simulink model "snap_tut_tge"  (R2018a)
settings: Solver=VariableStepDiscrete  StartTime=0.0  StopTime=50000  RelTol=1e-3
undefined symbols (not defined in the file): bad_frame, Bit, Both, bram, c, cnt_rst, core_rst, d, data, data_in, eof, eof_in, Falling, hex2dec, ip, ip_in, led, led_rx, led_tx, led_up, link_up, Location, Lower, Minimum_Area, notused, out, overrun, reg, Rising, ROACH2, sfp, SNAP, tx_full, tx_over, Unsigned, Upper, valid, valid_in, Width, xc7k160t
libraries: xbsIndex_r4 x1201, casper_library_misc x9, xps_library x5
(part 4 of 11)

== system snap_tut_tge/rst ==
  sim_1 : Inport
  sim_2 : Inport  Port=2
  convert1_1 : DataTypeConversion  OutDataTypeStr=fixdt('ufix1_En0')
  convert1_2 : DataTypeConversion  OutDataTypeStr=fixdt('ufix1_En0')
  convert2_1 : DataTypeConversion  OutDataTypeStr=fixdt('ufix1_En0')  ConvertRealWorld=Stored Integer (SI)
  convert2_2 : DataTypeConversion  OutDataTypeStr=fixdt('ufix1_En0')  ConvertRealWorld=Stored Integer (SI)
  gain_1 : Gain  Gain=2
  gain_2 : Gain
  io_delay : xbsIndex_r4/Delay  rst=off  infoeditControl=Selection of Reset will increase slice count due to use of real FFs and instead of SRLs  en=off  latency=0  reg_retiming=on  dbl_ovrd=off  block_type=delay
  sim_add : Sum  OutDataTypeStr=uint32
  slice_cnt_rst : xbsIndex_r4/Slice  nbits=1  boolean_output=on  mode=Lower Bit Location + Width  bit1=0  base1=MSB of Input  bit0=0  base0=LSB of Input  dbl_ovrd=off  block_type=slice
  slice_core_rst : xbsIndex_r4/Slice  nbits=1  boolean_output=on  mode=Lower Bit Location + Width  bit1=0  base1=MSB of Input  bit0=1  base0=LSB of Input  dbl_ovrd=off  block_type=slice
  snap_tut_tge_rst_user_data_out : xbsIndex_r4/Gateway In  gui_display_data_type=Fixed-point  arith_type=Unsigned  n_bits=32  bin_pt=0  preci_type=Single  exp_width=8  frac_width=24  rows=1  columns=1  quantization="Round  (unbiased: +/- Inf)"  overflow=Saturate  period=1  UseAsADC=off  ADCChannel='1'  interface=None  automatic_assignment=on  address_offset=hex2dec('00')  intf_name=''  intf_description=''  default_value=0  timing_constraint=None  locs_specified=off  LOCs={}  io_standard={}  inherit_from_input=off  hdl_port=on  dbl_ovrd=off  block_type=gatewayin
  in_core_rst : Outport
  in_cnt_rst : Outport  Port=2
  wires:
  snap_tut_tge_rst_user_data_out/1 -> io_delay/1
  sim_add/1 -> snap_tut_tge_rst_user_data_out/1
  sim_1/1 -> convert1_1/1
  convert1_1/1 -> convert2_1/1
  convert2_1/1 -> gain_1/1
  gain_1/1 -> sim_add/1
  io_delay/1 -> slice_core_rst/1, slice_cnt_rst/1
  slice_core_rst/1 -> in_core_rst/1
  sim_2/1 -> convert1_2/1
  convert1_2/1 -> convert2_2/1
  convert2_2/1 -> gain_2/1
  gain_2/1 -> sim_add/2
  slice_cnt_rst/1 -> in_cnt_rst/1

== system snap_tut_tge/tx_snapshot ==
  in_data : Inport
  in_valid : Inport  Port=2
  in_eof : Inport  Port=3
  we : Inport  Port=4
  trig : Inport  Port=5
  assert_data : xbsIndex_r4/Assert  assert_type=on  type_source=Explicitly  gui_display_data_type=Fixed-point  arith_type=Unsigned  n_bits=64  bin_pt=0  preci_type=Single  exp_width=8  frac_width=24  assert_rate=off  rate_source=Explicitly  period=1  output_port=on  block_type=assert
  assert_eof : xbsIndex_r4/Assert  assert_type=on  type_source=Explicitly  gui_display_data_type=Boolean  arith_type=Boolean  n_bits=1  bin_pt=0  preci_type=Single  exp_width=8  frac_width=24  assert_rate=off  rate_source=Explicitly  period=1  output_port=on  block_type=assert
  assert_valid : xbsIndex_r4/Assert  assert_type=on  type_source=Explicitly  gui_display_data_type=Boolean  arith_type=Boolean  n_bits=1  bin_pt=0  preci_type=Single  exp_width=8  frac_width=24  assert_rate=off  rate_source=Explicitly  period=1  output_port=on  block_type=assert
  buscreate : Subsystem  AncestorBlock=casper_library_flow_control/bus_create  mask(bus_create){inputNum=3}
      mask prompts: inputNum "Number of inputs:"
      mask init:
      | bus_create_init(gcb,...
      |     'inputNum', inputNum);
  ss : Subsystem  Tag=casper:snapshot  AncestorBlock=casper_library_scopes/snapshot  mask(snapshot){storage=bram, dram_dimm=2, dram_clock=250, nsamples=12, data_width=128, offset=off, circap=off, value=off, ext_arm=off, ext_circ=off, provide_outputs=off, use_dsp48=on}
      mask prompts: storage "Storage medium"; dram_dimm "DRAM dimm"; dram_clock "DRAM clock rate"; nsamples "Number of Samples (2^?)"; data_width "Data width"; offset "Start delay support"; circap "Circular capture support"; value "Extra value capture support"; ext_arm "External arm support"; ext_circ "External circular capture support"; provide_outputs "Provide outputs"; use_dsp48 "Use DSP48s to implement counters"
      mask help: Standard snap block, but with the following optional extras; 1) Optionally delay the fabric trigger by a user-specified number of valids. 2) Capture continuously after a trigger until a stop pulse is received. Data is captured into BRAM continuously, with old data being overwritten until a stop command is received. Then stop capturing when memory is filled. This enables you to get some data before and some data after the stop pulse. Use the 'tr_en_cnt' register to determine where you are in your vector. 'Addr' register's MSb now indicates 'busy capturing'. 3) Optionally capture a value on an i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
      mask init:
      | snapshot_init(gcb, ...
      |     'storage', storage, ...
      |     'dram_dimm', dram_dimm, ...
      |     'dram_clock', dram_clock, ...
      |     'nsamples', nsamples, ...
      |     'data_width', data_width, ...
      |     'offset', offset, ...
      |     'circap', circap, ...
      |     'value', value, ...
      |     'ext_arm', ext_arm, ...
      |     'ext_circ', ext_circ, ...
      |     'provide_outputs', 'off', ...
      |     'use_dsp48', use_dsp48);
  arm_out : Outport
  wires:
  ss/1(arm_out) -> arm_out/1
  buscreate/1(bus_out) -> ss/1(din)
  in_data/1 -> assert_data/1
  assert_data/1 -> buscreate/1(in1)
  in_valid/1 -> assert_valid/1
  assert_valid/1 -> buscreate/2(in2)
  in_eof/1 -> assert_eof/1
  assert_eof/1 -> buscreate/3(in3)
  we/1 -> ss/2(we)
  trig/1 -> ss/3(trig)

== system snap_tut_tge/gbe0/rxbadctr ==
  out_reg : Inport
  assert_reg : xbsIndex_r4/Assert  assert_type=on  type_source=Explicitly  gui_display_data_type=Fixed-point  arith_type=Unsigned  n_bits=32  bin_pt=0  preci_type=Single  exp_width=8  frac_width=24  assert_rate=off  rate_source=Explicitly  period=1  output_port=on  block_type=assert
  cast_gw : xbsIndex_r4/Convert  gui_display_data_type=Fixed-point  arith_type=Unsigned  n_bits=32  bin_pt=0  float_type=Single  exp_bits=8  fraction_bits=24  quantization=Truncate  overflow=Wrap  en=off  latency=1  pipeline=off  dbl_ovrd=off  block_type=convert
  io_delay : xbsIndex_r4/Delay  rst=off  infoeditControl=Selection of Reset will increase slice count due to use of real FFs and instead of SRLs  en=off  latency=1  reg_retiming=on  dbl_ovrd=off  block_type=delay
  reint1 : xbsIndex_r4/Reinterpret  force_arith_type=on  arith_type=Unsigned  force_bin_pt=on  bin_pt=0  block_type=reinterpret
  sim_out : Terminator
  snap_tut_tge_gbe0_rxbadctr_user_data_in : xbsIndex_r4/Gateway Out  inherit_from_input=off  hdl_port=on  rows=1  columns=1  UseAsDAC=off  DACChannel='1'  interface=None  automatic_assignment=on  address_offset=hex2dec('00')  intf_name=''  intf_description=''  timing_constraint=None  locs_specified=off  LOCs={}  io_standard={}  block_type=gatewayout
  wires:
  io_delay/1 -> cast_gw/1
  cast_gw/1 -> snap_tut_tge_gbe0_rxbadctr_user_data_in/1
  snap_tut_tge_gbe0_rxbadctr_user_data_in/1 -> sim_out/1
  out_reg/1 -> assert_reg/1
  assert_reg/1 -> reint1/1
  reint1/1 -> io_delay/1

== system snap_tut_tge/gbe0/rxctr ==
  out_reg : Inport
  assert_reg : xbsIndex_r4/Assert  assert_type=on  type_source=Explicitly  gui_display_data_type=Fixed-point  arith_type=Unsigned  n_bits=32  bin_pt=0  preci_type=Single  exp_width=8  frac_width=24  assert_rate=off  rate_source=Explicitly  period=1  output_port=on  block_type=assert
  cast_gw : xbsIndex_r4/Convert  gui_display_data_type=Fixed-point  arith_type=Unsigned  n_bits=32  bin_pt=0  float_type=Single  exp_bits=8  fraction_bits=24  quantization=Truncate  overflow=Wrap  en=off  latency=1  pipeline=off  dbl_ovrd=off  block_type=convert
  io_delay : xbsIndex_r4/Delay  rst=off  infoeditControl=Selection of Reset will increase slice count due to use of real FFs and instead of SRLs  en=off  latency=1  reg_retiming=on  dbl_ovrd=off  block_type=delay
  reint1 : xbsIndex_r4/Reinterpret  force_arith_type=on  arith_type=Unsigned  force_bin_pt=on  bin_pt=0  block_type=reinterpret
  sim_out : Terminator
  snap_tut_tge_gbe0_rxctr_user_data_in : xbsIndex_r4/Gateway Out  inherit_from_input=off  hdl_port=on  rows=1  columns=1  UseAsDAC=off  DACChannel='1'  interface=None  automatic_assignment=on  address_offset=hex2dec('00')  intf_name=''  intf_description=''  timing_constraint=None  locs_specified=off  LOCs={}  io_standard={}  block_type=gatewayout
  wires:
  io_delay/1 -> cast_gw/1
  cast_gw/1 -> snap_tut_tge_gbe0_rxctr_user_data_in/1
  snap_tut_tge_gbe0_rxctr_user_data_in/1 -> sim_out/1
  out_reg/1 -> assert_reg/1
  assert_reg/1 -> reint1/1
  reint1/1 -> io_delay/1

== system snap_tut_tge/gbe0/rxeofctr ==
  out_reg : Inport
  assert_reg : xbsIndex_r4/Assert  assert_type=on  type_source=Explicitly  gui_display_data_type=Fixed-point  arith_type=Unsigned  n_bits=32  bin_pt=0  preci_type=Single  exp_width=8  frac_width=24  assert_rate=off  rate_source=Explicitly  period=1  output_port=on  block_type=assert
  cast_gw : xbsIndex_r4/Convert  gui_display_data_type=Fixed-point  arith_type=Unsigned  n_bits=32  bin_pt=0  float_type=Single  exp_bits=8  fraction_bits=24  quantization=Truncate  overflow=Wrap  en=off  latency=1  pipeline=off  dbl_ovrd=off  block_type=convert
  io_delay : xbsIndex_r4/Delay  rst=off  infoeditControl=Selection of Reset will increase slice count due to use of real FFs and instead of SRLs  en=off  latency=1  reg_retiming=on  dbl_ovrd=off  block_type=delay
  reint1 : xbsIndex_r4/Reinterpret  force_arith_type=on  arith_type=Unsigned  force_bin_pt=on  bin_pt=0  block_type=reinterpret
  sim_out : Terminator
  snap_tut_tge_gbe0_rxeofctr_user_data_in : xbsIndex_r4/Gateway Out  inherit_from_input=off  hdl_port=on  rows=1  columns=1  UseAsDAC=off  DACChannel='1'  interface=None  automatic_assignment=on  address_offset=hex2dec('00')  intf_name=''  intf_description=''  timing_constraint=None  locs_specified=off  LOCs={}  io_standard={}  block_type=gatewayout
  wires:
  io_delay/1 -> cast_gw/1
  cast_gw/1 -> snap_tut_tge_gbe0_rxeofctr_user_data_in/1
  snap_tut_tge_gbe0_rxeofctr_user_data_in/1 -> sim_out/1
  out_reg/1 -> assert_reg/1
  assert_reg/1 -> reint1/1
  reint1/1 -> io_delay/1

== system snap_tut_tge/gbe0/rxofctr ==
  out_reg : Inport
  assert_reg : xbsIndex_r4/Assert  assert_type=on  type_source=Explicitly  gui_display_data_type=Fixed-point  arith_type=Unsigned  n_bits=32  bin_pt=0  preci_type=Single  exp_width=8  frac_width=24  assert_rate=off  rate_source=Explicitly  period=1  output_port=on  block_type=assert
  cast_gw : xbsIndex_r4/Convert  gui_display_data_type=Fixed-point  arith_type=Unsigned  n_bits=32  bin_pt=0  float_type=Single  exp_bits=8  fraction_bits=24  quantization=Truncate  overflow=Wrap  en=off  latency=1  pipeline=off  dbl_ovrd=off  block_type=convert
  io_delay : xbsIndex_r4/Delay  rst=off  infoeditControl=Selection of Reset will increase slice count due to use of real FFs and instead of SRLs  en=off  latency=1  reg_retiming=on  dbl_ovrd=off  block_type=delay
  reint1 : xbsIndex_r4/Reinterpret  force_arith_type=on  arith_type=Unsigned  force_bin_pt=on  bin_pt=0  block_type=reinterpret
  sim_out : Terminator
  snap_tut_tge_gbe0_rxofctr_user_data_in : xbsIndex_r4/Gateway Out  inherit_from_input=off  hdl_port=on  rows=1  columns=1  UseAsDAC=off  DACChannel='1'  interface=None  automatic_assignment=on  address_offset=hex2dec('00')  intf_name=''  intf_description=''  timing_constraint=None  locs_specified=off  LOCs={}  io_standard={}  block_type=gatewayout
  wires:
  io_delay/1 -> cast_gw/1
  cast_gw/1 -> snap_tut_tge_gbe0_rxofctr_user_data_in/1
  snap_tut_tge_gbe0_rxofctr_user_data_in/1 -> sim_out/1
  out_reg/1 -> assert_reg/1
  assert_reg/1 -> reint1/1
  reint1/1 -> io_delay/1

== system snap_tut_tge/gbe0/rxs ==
  in_led_up : Inport
  in_led_rx : Inport  Port=2
  in_data_in : Inport  Port=3
  in_valid_in : Inport  Port=4
  in_ip_in : Inport  Port=5
  in_eof_in : Inport  Port=6
  in_bad_frame : Inport  Port=7
  in_overrun : Inport  Port=8
  we : Inport  Port=9
  trig : Inport  Port=10
  assert_bad_frame : xbsIndex_r4/Assert  assert_type=on  type_source=Explicitly  gui_display_data_type=Boolean  arith_type=Boolean  n_bits=1  bin_pt=0  preci_type=Single  exp_width=8  frac_width=24  assert_rate=off  rate_source=Explicitly  period=1  output_port=on  block_type=assert
  assert_data_in : xbsIndex_r4/Assert  assert_type=on  type_source=Explicitly  gui_display_data_type=Fixed-point  arith_type=Unsigned  n_bits=64  bin_pt=0  preci_type=Single  exp_width=8  frac_width=24  assert_rate=off  rate_source=Explicitly  period=1  output_port=on  block_type=assert
  assert_eof_in : xbsIndex_r4/Assert  assert_type=on  type_source=Explicitly  gui_display_data_type=Boolean  arith_type=Boolean  n_bits=1  bin_pt=0  preci_type=Single  exp_width=8  frac_width=24  assert_rate=off  rate_source=Explicitly  period=1  output_port=on  block_type=assert
  assert_ip_in : xbsIndex_r4/Assert  assert_type=on  type_source=Explicitly  gui_display_data_type=Fixed-point  arith_type=Unsigned  n_bits=32  bin_pt=0  preci_type=Single  exp_width=8  frac_width=24  assert_rate=off  rate_source=Explicitly  period=1  output_port=on  block_type=assert
  assert_led_rx : xbsIndex_r4/Assert  assert_type=on  type_source=Explicitly  gui_display_data_type=Boolean  arith_type=Boolean  n_bits=1  bin_pt=0  preci_type=Single  exp_width=8  frac_width=24  assert_rate=off  rate_source=Explicitly  period=1  output_port=on  block_type=assert
  assert_led_up : xbsIndex_r4/Assert  assert_type=on  type_source=Explicitly  gui_display_data_type=Boolean  arith_type=Boolean  n_bits=1  bin_pt=0  preci_type=Single  exp_width=8  frac_width=24  assert_rate=off  rate_source=Explicitly  period=1  output_port=on  block_type=assert
  assert_overrun : xbsIndex_r4/Assert  assert_type=on  type_source=Explicitly  gui_display_data_type=Boolean  arith_type=Boolean  n_bits=1  bin_pt=0  preci_type=Single  exp_width=8  frac_width=24  assert_rate=off  rate_source=Explicitly  period=1  output_port=on  block_type=assert
  assert_valid_in : xbsIndex_r4/Assert  assert_type=on  type_source=Explicitly  gui_display_data_type=Boolean  arith_type=Boolean  n_bits=1  bin_pt=0  preci_type=Single  exp_width=8  frac_width=24  assert_rate=off  rate_source=Explicitly  period=1  output_port=on  block_type=assert
  buscreate : Subsystem  AncestorBlock=casper_library_flow_control/bus_create  mask(bus_create){inputNum=8}
      mask prompts: inputNum "Number of inputs:"
      mask init:
      | bus_create_init(gcb,...
      |     'inputNum', inputNum);
  io_delay : Subsystem  AncestorBlock=casper_library_delays/pipeline  mask(pipeline){csp_latency=5}
      mask prompts: csp_latency "Latency"
      mask help: An explicitly laid-out delay line to avoid mapping to SRL16s for use in pipelining to help achieve timing closure.
      mask init:
      | pipeline_init(gcb,'latency',csp_latency);
  ss : Subsystem  Tag=casper:snapshot  AncestorBlock=casper_library_scopes/snapshot  mask(snapshot){storage=bram, dram_dimm=2, dram_clock=250, nsamples=13, data_width=128, offset=off, circap=off, value=off, ext_arm=off, ext_circ=off, provide_outputs=off, use_dsp48=on}
      mask prompts: storage "Storage medium"; dram_dimm "DRAM dimm"; dram_clock "DRAM clock rate"; nsamples "Number of Samples (2^?)"; data_width "Data width"; offset "Start delay support"; circap "Circular capture support"; value "Extra value capture support"; ext_arm "External arm support"; ext_circ "External circular capture support"; provide_outputs "Provide outputs"; use_dsp48 "Use DSP48s to implement counters"
      mask help: Standard snap block, but with the following optional extras; 1) Optionally delay the fabric trigger by a user-specified number of valids. 2) Capture continuously after a trigger until a stop pulse is received. Data is captured into BRAM continuously, with old data being overwritten until a stop command is received. Then stop capturing when memory is filled. This enables you to get some data before and some data after the stop pulse. Use the 'tr_en_cnt' register to determine where you are in your vector. 'Addr' register's MSb now indicates 'busy capturing'. 3) Optionally capture a value on an i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
      mask init:
      | snapshot_init(gcb, ...
      |     'storage', storage, ...
      |     'dram_dimm', dram_dimm, ...
      |     'dram_clock', dram_clock, ...
      |     'nsamples', nsamples, ...
      |     'data_width', data_width, ...
      |     'offset', offset, ...
      |     'circap', circap, ...
      |     'value', value, ...
      |     'ext_arm', ext_arm, ...
      |     'ext_circ', ext_circ, ...
      |     'provide_outputs', 'off', ...
      |     'use_dsp48', use_dsp48);
  trig_delay : Subsystem  AncestorBlock=casper_library_delays/pipeline  mask(pipeline){csp_latency=5}
      mask prompts: csp_latency "Latency"
      mask help: An explicitly laid-out delay line to avoid mapping to SRL16s for use in pipelining to help achieve timing closure.
      mask init:
      | pipeline_init(gcb,'latency',csp_latency);
  we_delay : Subsystem  AncestorBlock=casper_library_delays/pipeline  mask(pipeline){csp_latency=5}
      mask prompts: csp_latency "Latency"
      mask help: An explicitly laid-out delay line to avoid mapping to SRL16s for use in pipelining to help achieve timing closure.
      mask init:
      | pipeline_init(gcb,'latency',csp_latency);
  arm_out : Outport
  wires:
  ss/1(arm_out) -> arm_out/1
  buscreate/1(bus_out) -> io_delay/1(d)
  io_delay/1(q) -> ss/1(din)
  in_led_up/1 -> assert_led_up/1
  assert_led_up/1 -> buscreate/1(in1)
  in_led_rx/1 -> assert_led_rx/1
  assert_led_rx/1 -> buscreate/2(in2)
  in_data_in/1 -> assert_data_in/1
  assert_data_in/1 -> buscreate/3(in3)
  in_valid_in/1 -> assert_valid_in/1
  assert_valid_in/1 -> buscreate/4(in4)
  in_ip_in/1 -> assert_ip_in/1
  assert_ip_in/1 -> buscreate/5(in5)
  in_eof_in/1 -> assert_eof_in/1
  assert_eof_in/1 -> buscreate/6(in6)
  in_bad_frame/1 -> assert_bad_frame/1
  assert_bad_frame/1 -> buscreate/7(in7)
  in_overrun/1 -> assert_overrun/1
  assert_overrun/1 -> buscreate/8(in8)
  we/1 -> we_delay/1(d)
  we_delay/1(q) -> ss/2(we)
  trig/1 -> trig_delay/1(d)
  trig_delay/1(q) -> ss/3(trig)

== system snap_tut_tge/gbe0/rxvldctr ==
  out_reg : Inport
  assert_reg : xbsIndex_r4/Assert  assert_type=on  type_source=Explicitly  gui_display_data_type=Fixed-point  arith_type=Unsigned  n_bits=32  bin_pt=0  preci_type=Single  exp_width=8  frac_width=24  assert_rate=off  rate_source=Explicitly  period=1  output_port=on  block_type=assert
  cast_gw : xbsIndex_r4/Convert  gui_display_data_type=Fixed-point  arith_type=Unsigned  n_bits=32  bin_pt=0  float_type=Single  exp_bits=8  fraction_bits=24  quantization=Truncate  overflow=Wrap  en=off  latency=1  pipeline=off  dbl_ovrd=off  block_type=convert
  io_delay : xbsIndex_r4/Delay  rst=off  infoeditControl=Selection of Reset will increase slice count due to use of real FFs and instead of SRLs  en=off  latency=1  reg_retiming=on  dbl_ovrd=off  block_type=delay
  reint1 : xbsIndex_r4/Reinterpret  force_arith_type=on  arith_type=Unsigned  force_bin_pt=on  bin_pt=0  block_type=reinterpret
  sim_out : Terminator
  snap_tut_tge_gbe0_rxvldctr_user_data_in : xbsIndex_r4/Gateway Out  inherit_from_input=off  hdl_port=on  rows=1  columns=1  UseAsDAC=off  DACChannel='1'  interface=None  automatic_assignment=on  address_offset=hex2dec('00')  intf_name=''  intf_description=''  timing_constraint=None  locs_specified=off  LOCs={}  io_standard={}  block_type=gatewayout
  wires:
  io_delay/1 -> cast_gw/1
  cast_gw/1 -> snap_tut_tge_gbe0_rxvldctr_user_data_in/1
  snap_tut_tge_gbe0_rxvldctr_user_data_in/1 -> sim_out/1
  out_reg/1 -> assert_reg/1
  assert_reg/1 -> reint1/1
  reint1/1 -> io_delay/1

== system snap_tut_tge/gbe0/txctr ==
  out_reg : Inport
  assert_reg : xbsIndex_r4/Assert  assert_type=on  type_source=Explicitly  gui_display_data_type=Fixed-point  arith_type=Unsigned  n_bits=32  bin_pt=0  preci_type=Single  exp_width=8  frac_width=24  assert_rate=off  rate_source=Explicitly  period=1  output_port=on  block_type=assert
  cast_gw : xbsIndex_r4/Convert  gui_display_data_type=Fixed-point  arith_type=Unsigned  n_bits=32  bin_pt=0  float_type=Single  exp_bits=8  fraction_bits=24  quantization=Truncate  overflow=Wrap  en=off  latency=1  pipeline=off  dbl_ovrd=off  block_type=convert
  io_delay : xbsIndex_r4/Delay  rst=off  infoeditControl=Selection of Reset will increase slice count due to use of real FFs and instead of SRLs  en=off  latency=1  reg_retiming=on  dbl_ovrd=off  block_type=delay
  reint1 : xbsIndex_r4/Reinterpret  force_arith_type=on  arith_type=Unsigned  force_bin_pt=on  bin_pt=0  block_type=reinterpret
  sim_out : Terminator
  snap_tut_tge_gbe0_txctr_user_data_in : xbsIndex_r4/Gateway Out  inherit_from_input=off  hdl_port=on  rows=1  columns=1  UseAsDAC=off  DACChannel='1'  interface=None  automatic_assignment=on  address_offset=hex2dec('00')  intf_name=''  intf_description=''  timing_constraint=None  locs_specified=off  LOCs={}  io_standard={}  block_type=gatewayout
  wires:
  io_delay/1 -> cast_gw/1
  cast_gw/1 -> snap_tut_tge_gbe0_txctr_user_data_in/1
  snap_tut_tge_gbe0_txctr_user_data_in/1 -> sim_out/1
  out_reg/1 -> assert_reg/1
  assert_reg/1 -> reint1/1
  reint1/1 -> io_delay/1

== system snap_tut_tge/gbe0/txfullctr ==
  out_reg : Inport
  assert_reg : xbsIndex_r4/Assert  assert_type=on  type_source=Explicitly  gui_display_data_type=Fixed-point  arith_type=Unsigned  n_bits=32  bin_pt=0  preci_type=Single  exp_width=8  frac_width=24  assert_rate=off  rate_source=Explicitly  period=1  output_port=on  block_type=assert
  cast_gw : xbsIndex_r4/Convert  gui_display_data_type=Fixed-point  arith_type=Unsigned  n_bits=32  bin_pt=0  float_type=Single  exp_bits=8  fraction_bits=24  quantization=Truncate  overflow=Wrap  en=off  latency=1  pipeline=off  dbl_ovrd=off  block_type=convert
  io_delay : xbsIndex_r4/Delay  rst=off  infoeditControl=Selection of Reset will increase slice count due to use of real FFs and instead of SRLs  en=off  latency=1  reg_retiming=on  dbl_ovrd=off  block_type=delay
  reint1 : xbsIndex_r4/Reinterpret  force_arith_type=on  arith_type=Unsigned  force_bin_pt=on  bin_pt=0  block_type=reinterpret
  sim_out : Terminator
  snap_tut_tge_gbe0_txfullctr_user_data_in : xbsIndex_r4/Gateway Out  inherit_from_input=off  hdl_port=on  rows=1  columns=1  UseAsDAC=off  DACChannel='1'  interface=None  automatic_assignment=on  address_offset=hex2dec('00')  intf_name=''  intf_description=''  timing_constraint=None  locs_specified=off  LOCs={}  io_standard={}  block_type=gatewayout
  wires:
  io_delay/1 -> cast_gw/1
  cast_gw/1 -> snap_tut_tge_gbe0_txfullctr_user_data_in/1
  snap_tut_tge_gbe0_txfullctr_user_data_in/1 -> sim_out/1
  out_reg/1 -> assert_reg/1
  assert_reg/1 -> reint1/1
  reint1/1 -> io_delay/1

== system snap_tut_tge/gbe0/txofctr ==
  out_reg : Inport
  assert_reg : xbsIndex_r4/Assert  assert_type=on  type_source=Explicitly  gui_display_data_type=Fixed-point  arith_type=Unsigned  n_bits=32  bin_pt=0  preci_type=Single  exp_width=8  frac_width=24  assert_rate=off  rate_source=Explicitly  period=1  output_port=on  block_type=assert
  cast_gw : xbsIndex_r4/Convert  gui_display_data_type=Fixed-point  arith_type=Unsigned  n_bits=32  bin_pt=0  float_type=Single  exp_bits=8  fraction_bits=24  quantization=Truncate  overflow=Wrap  en=off  latency=1  pipeline=off  dbl_ovrd=off  block_type=convert
  io_delay : xbsIndex_r4/Delay  rst=off  infoeditControl=Selection of Reset will increase slice count due to use of real FFs and instead of SRLs  en=off  latency=1  reg_retiming=on  dbl_ovrd=off  block_type=delay
  reint1 : xbsIndex_r4/Reinterpret  force_arith_type=on  arith_type=Unsigned  force_bin_pt=on  bin_pt=0  block_type=reinterpret
  sim_out : Terminator
  snap_tut_tge_gbe0_txofctr_user_data_in : xbsIndex_r4/Gateway Out  inherit_from_input=off  hdl_port=on  rows=1  columns=1  UseAsDAC=off  DACChannel='1'  interface=None  automatic_assignment=on  address_offset=hex2dec('00')  intf_name=''  intf_description=''  timing_constraint=None  locs_specified=off  LOCs={}  io_standard={}  block_type=gatewayout
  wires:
  io_delay/1 -> cast_gw/1
  cast_gw/1 -> snap_tut_tge_gbe0_txofctr_user_data_in/1
  snap_tut_tge_gbe0_txofctr_user_data_in/1 -> sim_out/1
  out_reg/1 -> assert_reg/1
  assert_reg/1 -> reint1/1
  reint1/1 -> io_delay/1

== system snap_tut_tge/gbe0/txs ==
  in_link_up : Inport
  in_led_tx : Inport  Port=2
  in_tx_full : Inport  Port=3
  in_tx_over : Inport  Port=4
  in_valid : Inport  Port=5
  in_eof : Inport  Port=6
  in_data : Inport  Port=7
  in_ip : Inport  Port=8
  we : Inport  Port=9
  trig : Inport  Port=10
  assert_data : xbsIndex_r4/Assert  assert_type=on  type_source=Explicitly  gui_display_data_type=Fixed-point  arith_type=Unsigned  n_bits=64  bin_pt=0  preci_type=Single  exp_width=8  frac_width=24  assert_rate=off  rate_source=Explicitly  period=1  output_port=on  block_type=assert
  assert_eof : xbsIndex_r4/Assert  assert_type=on  type_source=Explicitly  gui_display_data_type=Boolean  arith_type=Boolean  n_bits=1  bin_pt=0  preci_type=Single  exp_width=8  frac_width=24  assert_rate=off  rate_source=Explicitly  period=1  output_port=on  block_type=assert
  assert_ip : xbsIndex_r4/Assert  assert_type=on  type_source=Explicitly  gui_display_data_type=Fixed-point  arith_type=Unsigned  n_bits=32  bin_pt=0  preci_type=Single  exp_width=8  frac_width=24  assert_rate=off  rate_source=Explicitly  period=1  output_port=on  block_type=assert
  assert_led_tx : xbsIndex_r4/Assert  assert_type=on  type_source=Explicitly  gui_display_data_type=Boolean  arith_type=Boolean  n_bits=1  bin_pt=0  preci_type=Single  exp_width=8  frac_width=24  assert_rate=off  rate_source=Explicitly  period=1  output_port=on  block_type=assert
  assert_link_up : xbsIndex_r4/Assert  assert_type=on  type_source=Explicitly  gui_display_data_type=Boolean  arith_type=Boolean  n_bits=1  bin_pt=0  preci_type=Single  exp_width=8  frac_width=24  assert_rate=off  rate_source=Explicitly  period=1  output_port=on  block_type=assert
  assert_tx_full : xbsIndex_r4/Assert  assert_type=on  type_source=Explicitly  gui_display_data_type=Boolean  arith_type=Boolean  n_bits=1  bin_pt=0  preci_type=Single  exp_width=8  frac_width=24  assert_rate=off  rate_source=Explicitly  period=1  output_port=on  block_type=assert
  assert_tx_over : xbsIndex_r4/Assert  assert_type=on  type_source=Explicitly  gui_display_data_type=Boolean  arith_type=Boolean  n_bits=1  bin_pt=0  preci_type=Single  exp_width=8  frac_width=24  assert_rate=off  rate_source=Explicitly  period=1  output_port=on  block_type=assert
  assert_valid : xbsIndex_r4/Assert  assert_type=on  type_source=Explicitly  gui_display_data_type=Boolean  arith_type=Boolean  n_bits=1  bin_pt=0  preci_type=Single  exp_width=8  frac_width=24  assert_rate=off  rate_source=Explicitly  period=1  output_port=on  block_type=assert
  buscreate : Subsystem  AncestorBlock=casper_library_flow_control/bus_create  mask(bus_create){inputNum=8}
      mask prompts: inputNum "Number of inputs:"
      mask init:
      | bus_create_init(gcb,...
      |     'inputNum', inputNum);
  io_delay : Subsystem  AncestorBlock=casper_library_delays/pipeline  mask(pipeline){csp_latency=5}
      mask prompts: csp_latency "Latency"
      mask help: An explicitly laid-out delay line to avoid mapping to SRL16s for use in pipelining to help achieve timing closure.
      mask init:
      | pipeline_init(gcb,'latency',csp_latency);
  ss : Subsystem  Tag=casper:snapshot  AncestorBlock=casper_library_scopes/snapshot  mask(snapshot){storage=bram, dram_dimm=2, dram_clock=250, nsamples=13, data_width=128, offset=off, circap=off, value=off, ext_arm=off, ext_circ=off, provide_outputs=off, use_dsp48=on}
      mask prompts: storage "Storage medium"; dram_dimm "DRAM dimm"; dram_clock "DRAM clock rate"; nsamples "Number of Samples (2^?)"; data_width "Data width"; offset "Start delay support"; circap "Circular capture support"; value "Extra value capture support"; ext_arm "External arm support"; ext_circ "External circular capture support"; provide_outputs "Provide outputs"; use_dsp48 "Use DSP48s to implement counters"
      mask help: Standard snap block, but with the following optional extras; 1) Optionally delay the fabric trigger by a user-specified number of valids. 2) Capture continuously after a trigger until a stop pulse is received. Data is captured into BRAM continuously, with old data being overwritten until a stop command is received. Then stop capturing when memory is filled. This enables you to get some data before and some data after the stop pulse. Use the 'tr_en_cnt' register to determine where you are in your vector. 'Addr' register's MSb now indicates 'busy capturing'. 3) Optionally capture a value on an i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
      mask init:
      | snapshot_init(gcb, ...
      |     'storage', storage, ...
      |     'dram_dimm', dram_dimm, ...
      |     'dram_clock', dram_clock, ...
      |     'nsamples', nsamples, ...
      |     'data_width', data_width, ...
      |     'offset', offset, ...
      |     'circap', circap, ...
      |     'value', value, ...
      |     'ext_arm', ext_arm, ...
      |     'ext_circ', ext_circ, ...
      |     'provide_outputs', 'off', ...
      |     'use_dsp48', use_dsp48);
  trig_delay : Subsystem  AncestorBlock=casper_library_delays/pipeline  mask(pipeline){csp_latency=5}
      mask prompts: csp_latency "Latency"
      mask help: An explicitly laid-out delay line to avoid mapping to SRL16s for use in pipelining to help achieve timing closure.
      mask init:
      | pipeline_init(gcb,'latency',csp_latency);
  we_delay : Subsystem  AncestorBlock=casper_library_delays/pipeline  mask(pipeline){csp_latency=5}
      mask prompts: csp_latency "Latency"
      mask help: An explicitly laid-out delay line to avoid mapping to SRL16s for use in pipelining to help achieve timing closure.
      mask init:
      | pipeline_init(gcb,'latency',csp_latency);
  arm_out : Outport
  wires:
  ss/1(arm_out) -> arm_out/1
  buscreate/1(bus_out) -> io_delay/1(d)
  io_delay/1(q) -> ss/1(din)
  in_link_up/1 -> assert_link_up/1
  assert_link_up/1 -> buscreate/1(in1)
  in_led_tx/1 -> assert_led_tx/1
  assert_led_tx/1 -> buscreate/2(in2)
  in_tx_full/1 -> assert_tx_full/1
  assert_tx_full/1 -> buscreate/3(in3)
  in_tx_over/1 -> assert_tx_over/1
  assert_tx_over/1 -> buscreate/4(in4)
  in_valid/1 -> assert_valid/1
  assert_valid/1 -> buscreate/5(in5)
  in_eof/1 -> assert_eof/1
  assert_eof/1 -> buscreate/6(in6)
  in_data/1 -> assert_data/1
  assert_data/1 -> buscreate/7(in7)
  in_ip/1 -> assert_ip/1
  assert_ip/1 -> buscreate/8(in8)
  we/1 -> we_delay/1(d)
  we_delay/1(q) -> ss/2(we)
  trig/1 -> trig_delay/1(d)
  trig_delay/1(q) -> ss/3(trig)

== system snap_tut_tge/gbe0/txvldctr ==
  out_reg : Inport
  assert_reg : xbsIndex_r4/Assert  assert_type=on  type_source=Explicitly  gui_display_data_type=Fixed-point  arith_type=Unsigned  n_bits=32  bin_pt=0  preci_type=Single  exp_width=8  frac_width=24  assert_rate=off  rate_source=Explicitly  period=1  output_port=on  block_type=assert
  cast_gw : xbsIndex_r4/Convert  gui_display_data_type=Fixed-point  arith_type=Unsigned  n_bits=32  bin_pt=0  float_type=Single  exp_bits=8  fraction_bits=24  quantization=Truncate  overflow=Wrap  en=off  latency=1  pipeline=off  dbl_ovrd=off  block_type=convert
  io_delay : xbsIndex_r4/Delay  rst=off  infoeditControl=Selection of Reset will increase slice count due to use of real FFs and instead of SRLs  en=off  latency=1  reg_retiming=on  dbl_ovrd=off  block_type=delay
  reint1 : xbsIndex_r4/Reinterpret  force_arith_type=on  arith_type=Unsigned  force_bin_pt=on  bin_pt=0  block_type=reinterpret
  sim_out : Terminator
  snap_tut_tge_gbe0_txvldctr_user_data_in : xbsIndex_r4/Gateway Out  inherit_from_input=off  hdl_port=on  rows=1  columns=1  UseAsDAC=off  DACChannel='1'  interface=None  automatic_assignment=on  address_offset=hex2dec('00')  intf_name=''  intf_description=''  timing_constraint=None  locs_specified=off  LOCs={}  io_standard={}  block_type=gatewayout
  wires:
  io_delay/1 -> cast_gw/1
  cast_gw/1 -> snap_tut_tge_gbe0_txvldctr_user_data_in/1
  snap_tut_tge_gbe0_txvldctr_user_data_in/1 -> sim_out/1
  out_reg/1 -> assert_reg/1
  assert_reg/1 -> reint1/1
  reint1/1 -> io_delay/1

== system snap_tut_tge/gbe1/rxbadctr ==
  out_reg : Inport
  assert_reg : xbsIndex_r4/Assert  assert_type=on  type_source=Explicitly  gui_display_data_type=Fixed-point  arith_type=Unsigned  n_bits=32  bin_pt=0  preci_type=Single  exp_width=8  frac_width=24  assert_rate=off  rate_source=Explicitly  period=1  output_port=on  block_type=assert
  cast_gw : xbsIndex_r4/Convert  gui_display_data_type=Fixed-point  arith_type=Unsigned  n_bits=32  bin_pt=0  float_type=Single  exp_bits=8  fraction_bits=24  quantization=Truncate  overflow=Wrap  en=off  latency=1  pipeline=off  dbl_ovrd=off  block_type=convert
  io_delay : xbsIndex_r4/Delay  rst=off  infoeditControl=Selection of Reset will increase slice count due to use of real FFs and instead of SRLs  en=off  latency=1  reg_retiming=on  dbl_ovrd=off  block_type=delay
  reint1 : xbsIndex_r4/Reinterpret  force_arith_type=on  arith_type=Unsigned  force_bin_pt=on  bin_pt=0  block_type=reinterpret
  sim_out : Terminator
  snap_tut_tge_gbe1_rxbadctr_user_data_in : xbsIndex_r4/Gateway Out  inherit_from_input=off  hdl_port=on  rows=1  columns=1  UseAsDAC=off  DACChannel='1'  interface=None  automatic_assignment=on  address_offset=hex2dec('00')  intf_name=''  intf_description=''  timing_constraint=None  locs_specified=off  LOCs={}  io_standard={}  block_type=gatewayout
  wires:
  io_delay/1 -> cast_gw/1
  cast_gw/1 -> snap_tut_tge_gbe1_rxbadctr_user_data_in/1
  snap_tut_tge_gbe1_rxbadctr_user_data_in/1 -> sim_out/1
  out_reg/1 -> assert_reg/1
  assert_reg/1 -> reint1/1
  reint1/1 -> io_delay/1

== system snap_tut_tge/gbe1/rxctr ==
  out_reg : Inport
  assert_reg : xbsIndex_r4/Assert  assert_type=on  type_source=Explicitly  gui_display_data_type=Fixed-point  arith_type=Unsigned  n_bits=32  bin_pt=0  preci_type=Single  exp_width=8  frac_width=24  assert_rate=off  rate_source=Explicitly  period=1  output_port=on  block_type=assert
  cast_gw : xbsIndex_r4/Convert  gui_display_data_type=Fixed-point  arith_type=Unsigned  n_bits=32  bin_pt=0  float_type=Single  exp_bits=8  fraction_bits=24  quantization=Truncate  overflow=Wrap  en=off  latency=1  pipeline=off  dbl_ovrd=off  block_type=convert
  io_delay : xbsIndex_r4/Delay  rst=off  infoeditControl=Selection of Reset will increase slice count due to use of real FFs and instead of SRLs  en=off  latency=1  reg_retiming=on  dbl_ovrd=off  block_type=delay
  reint1 : xbsIndex_r4/Reinterpret  force_arith_type=on  arith_type=Unsigned  force_bin_pt=on  bin_pt=0  block_type=reinterpret
  sim_out : Terminator
  snap_tut_tge_gbe1_rxctr_user_data_in : xbsIndex_r4/Gateway Out  inherit_from_input=off  hdl_port=on  rows=1  columns=1  UseAsDAC=off  DACChannel='1'  interface=None  automatic_assignment=on  address_offset=hex2dec('00')  intf_name=''  intf_description=''  timing_constraint=None  locs_specified=off  LOCs={}  io_standard={}  block_type=gatewayout
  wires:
  io_delay/1 -> cast_gw/1
  cast_gw/1 -> snap_tut_tge_gbe1_rxctr_user_data_in/1
  snap_tut_tge_gbe1_rxctr_user_data_in/1 -> sim_out/1
  out_reg/1 -> assert_reg/1
  assert_reg/1 -> reint1/1
  reint1/1 -> io_delay/1

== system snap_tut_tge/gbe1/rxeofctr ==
  out_reg : Inport
  assert_reg : xbsIndex_r4/Assert  assert_type=on  type_source=Explicitly  gui_display_data_type=Fixed-point  arith_type=Unsigned  n_bits=32  bin_pt=0  preci_type=Single  exp_width=8  frac_width=24  assert_rate=off  rate_source=Explicitly  period=1  output_port=on  block_type=assert
  cast_gw : xbsIndex_r4/Convert  gui_display_data_type=Fixed-point  arith_type=Unsigned  n_bits=32  bin_pt=0  float_type=Single  exp_bits=8  fraction_bits=24  quantization=Truncate  overflow=Wrap  en=off  latency=1  pipeline=off  dbl_ovrd=off  block_type=convert
  io_delay : xbsIndex_r4/Delay  rst=off  infoeditControl=Selection of Reset will increase slice count due to use of real FFs and instead of SRLs  en=off  latency=1  reg_retiming=on  dbl_ovrd=off  block_type=delay
  reint1 : xbsIndex_r4/Reinterpret  force_arith_type=on  arith_type=Unsigned  force_bin_pt=on  bin_pt=0  block_type=reinterpret
  sim_out : Terminator
  snap_tut_tge_gbe1_rxeofctr_user_data_in : xbsIndex_r4/Gateway Out  inherit_from_input=off  hdl_port=on  rows=1  columns=1  UseAsDAC=off  DACChannel='1'  interface=None  automatic_assignment=on  address_offset=hex2dec('00')  intf_name=''  intf_description=''  timing_constraint=None  locs_specified=off  LOCs={}  io_standard={}  block_type=gatewayout
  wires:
  io_delay/1 -> cast_gw/1
  cast_gw/1 -> snap_tut_tge_gbe1_rxeofctr_user_data_in/1
  snap_tut_tge_gbe1_rxeofctr_user_data_in/1 -> sim_out/1
  out_reg/1 -> assert_reg/1
  assert_reg/1 -> reint1/1
  reint1/1 -> io_delay/1

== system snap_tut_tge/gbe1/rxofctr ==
  out_reg : Inport
  assert_reg : xbsIndex_r4/Assert  assert_type=on  type_source=Explicitly  gui_display_data_type=Fixed-point  arith_type=Unsigned  n_bits=32  bin_pt=0  preci_type=Single  exp_width=8  frac_width=24  assert_rate=off  rate_source=Explicitly  period=1  output_port=on  block_type=assert
  cast_gw : xbsIndex_r4/Convert  gui_display_data_type=Fixed-point  arith_type=Unsigned  n_bits=32  bin_pt=0  float_type=Single  exp_bits=8  fraction_bits=24  quantization=Truncate  overflow=Wrap  en=off  latency=1  pipeline=off  dbl_ovrd=off  block_type=convert
  io_delay : xbsIndex_r4/Delay  rst=off  infoeditControl=Selection of Reset will increase slice count due to use of real FFs and instead of SRLs  en=off  latency=1  reg_retiming=on  dbl_ovrd=off  block_type=delay
  reint1 : xbsIndex_r4/Reinterpret  force_arith_type=on  arith_type=Unsigned  force_bin_pt=on  bin_pt=0  block_type=reinterpret
  sim_out : Terminator
  snap_tut_tge_gbe1_rxofctr_user_data_in : xbsIndex_r4/Gateway Out  inherit_from_input=off  hdl_port=on  rows=1  columns=1  UseAsDAC=off  DACChannel='1'  interface=None  automatic_assignment=on  address_offset=hex2dec('00')  intf_name=''  intf_description=''  timing_constraint=None  locs_specified=off  LOCs={}  io_standard={}  block_type=gatewayout
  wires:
  io_delay/1 -> cast_gw/1
  cast_gw/1 -> snap_tut_tge_gbe1_rxofctr_user_data_in/1
  snap_tut_tge_gbe1_rxofctr_user_data_in/1 -> sim_out/1
  out_reg/1 -> assert_reg/1
  assert_reg/1 -> reint1/1
  reint1/1 -> io_delay/1

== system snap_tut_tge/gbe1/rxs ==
  in_led_up : Inport
  in_led_rx : Inport  Port=2
  in_data_in : Inport  Port=3
  in_valid_in : Inport  Port=4
  in_ip_in : Inport  Port=5
  in_eof_in : Inport  Port=6
  in_bad_frame : Inport  Port=7
  in_overrun : Inport  Port=8
  we : Inport  Port=9
  trig : Inport  Port=10
  assert_bad_frame : xbsIndex_r4/Assert  assert_type=on  type_source=Explicitly  gui_display_data_type=Boolean  arith_type=Boolean  n_bits=1  bin_pt=0  preci_type=Single  exp_width=8  frac_width=24  assert_rate=off  rate_source=Explicitly  period=1  output_port=on  block_type=assert
  assert_data_in : xbsIndex_r4/Assert  assert_type=on  type_source=Explicitly  gui_display_data_type=Fixed-point  arith_type=Unsigned  n_bits=64  bin_pt=0  preci_type=Single  exp_width=8  frac_width=24  assert_rate=off  rate_source=Explicitly  period=1  output_port=on  block_type=assert
  assert_eof_in : xbsIndex_r4/Assert  assert_type=on  type_source=Explicitly  gui_display_data_type=Boolean  arith_type=Boolean  n_bits=1  bin_pt=0  preci_type=Single  exp_width=8  frac_width=24  assert_rate=off  rate_source=Explicitly  period=1  output_port=on  block_type=assert
  assert_ip_in : xbsIndex_r4/Assert  assert_type=on  type_source=Explicitly  gui_display_data_type=Fixed-point  arith_type=Unsigned  n_bits=32  bin_pt=0  preci_type=Single  exp_width=8  frac_width=24  assert_rate=off  rate_source=Explicitly  period=1  output_port=on  block_type=assert
  assert_led_rx : xbsIndex_r4/Assert  assert_type=on  type_source=Explicitly  gui_display_data_type=Boolean  arith_type=Boolean  n_bits=1  bin_pt=0  preci_type=Single  exp_width=8  frac_width=24  assert_rate=off  rate_source=Explicitly  period=1  output_port=on  block_type=assert
  assert_led_up : xbsIndex_r4/Assert  assert_type=on  type_source=Explicitly  gui_display_data_type=Boolean  arith_type=Boolean  n_bits=1  bin_pt=0  preci_type=Single  exp_width=8  frac_width=24  assert_rate=off  rate_source=Explicitly  period=1  output_port=on  block_type=assert
  assert_overrun : xbsIndex_r4/Assert  assert_type=on  type_source=Explicitly  gui_display_data_type=Boolean  arith_type=Boolean  n_bits=1  bin_pt=0  preci_type=Single  exp_width=8  frac_width=24  assert_rate=off  rate_source=Explicitly  period=1  output_port=on  block_type=assert
  assert_valid_in : xbsIndex_r4/Assert  assert_type=on  type_source=Explicitly  gui_display_data_type=Boolean  arith_type=Boolean  n_bits=1  bin_pt=0  preci_type=Single  exp_width=8  frac_width=24  assert_rate=off  rate_source=Explicitly  period=1  output_port=on  block_type=assert
  buscreate : Subsystem  AncestorBlock=casper_library_flow_control/bus_create  mask(bus_create){inputNum=8}
      mask prompts: inputNum "Number of inputs:"
      mask init:
      | bus_create_init(gcb,...
      |     'inputNum', inputNum);
  io_delay : Subsystem  AncestorBlock=casper_library_delays/pipeline  mask(pipeline){csp_latency=5}
      mask prompts: csp_latency "Latency"
      mask help: An explicitly laid-out delay line to avoid mapping to SRL16s for use in pipelining to help achieve timing closure.
      mask init:
      | pipeline_init(gcb,'latency',csp_latency);
  ss : Subsystem  Tag=casper:snapshot  AncestorBlock=casper_library_scopes/snapshot  mask(snapshot){storage=bram, dram_dimm=2, dram_clock=250, nsamples=13, data_width=128, offset=off, circap=off, value=off, ext_arm=off, ext_circ=off, provide_outputs=off, use_dsp48=on}
      mask prompts: storage "Storage medium"; dram_dimm "DRAM dimm"; dram_clock "DRAM clock rate"; nsamples "Number of Samples (2^?)"; data_width "Data width"; offset "Start delay support"; circap "Circular capture support"; value "Extra value capture support"; ext_arm "External arm support"; ext_circ "External circular capture support"; provide_outputs "Provide outputs"; use_dsp48 "Use DSP48s to implement counters"
      mask help: Standard snap block, but with the following optional extras; 1) Optionally delay the fabric trigger by a user-specified number of valids. 2) Capture continuously after a trigger until a stop pulse is received. Data is captured into BRAM continuously, with old data being overwritten until a stop command is received. Then stop capturing when memory is filled. This enables you to get some data before and some data after the stop pulse. Use the 'tr_en_cnt' register to determine where you are in your vector. 'Addr' register's MSb now indicates 'busy capturing'. 3) Optionally capture a value on an i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
      mask init:
      | snapshot_init(gcb, ...
      |     'storage', storage, ...
      |     'dram_dimm', dram_dimm, ...
      |     'dram_clock', dram_clock, ...
      |     'nsamples', nsamples, ...
      |     'data_width', data_width, ...
      |     'offset', offset, ...
      |     'circap', circap, ...
      |     'value', value, ...
      |     'ext_arm', ext_arm, ...
      |     'ext_circ', ext_circ, ...
      |     'provide_outputs', 'off', ...
      |     'use_dsp48', use_dsp48);
  trig_delay : Subsystem  AncestorBlock=casper_library_delays/pipeline  mask(pipeline){csp_latency=5}
      mask prompts: csp_latency "Latency"
      mask help: An explicitly laid-out delay line to avoid mapping to SRL16s for use in pipelining to help achieve timing closure.
      mask init:
      | pipeline_init(gcb,'latency',csp_latency);
  we_delay : Subsystem  AncestorBlock=casper_library_delays/pipeline  mask(pipeline){csp_latency=5}
      mask prompts: csp_latency "Latency"
      mask help: An explicitly laid-out delay line to avoid mapping to SRL16s for use in pipelining to help achieve timing closure.
      mask init:
      | pipeline_init(gcb,'latency',csp_latency);
  arm_out : Outport
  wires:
  ss/1(arm_out) -> arm_out/1
  buscreate/1(bus_out) -> io_delay/1(d)
  io_delay/1(q) -> ss/1(din)
  in_led_up/1 -> assert_led_up/1
  assert_led_up/1 -> buscreate/1(in1)
  in_led_rx/1 -> assert_led_rx/1
  assert_led_rx/1 -> buscreate/2(in2)
  in_data_in/1 -> assert_data_in/1
  assert_data_in/1 -> buscreate/3(in3)
  in_valid_in/1 -> assert_valid_in/1
  assert_valid_in/1 -> buscreate/4(in4)
  in_ip_in/1 -> assert_ip_in/1
  assert_ip_in/1 -> buscreate/5(in5)
  in_eof_in/1 -> assert_eof_in/1
  assert_eof_in/1 -> buscreate/6(in6)
  in_bad_frame/1 -> assert_bad_frame/1
  assert_bad_frame/1 -> buscreate/7(in7)
  in_overrun/1 -> assert_overrun/1
  assert_overrun/1 -> buscreate/8(in8)
  we/1 -> we_delay/1(d)
  we_delay/1(q) -> ss/2(we)
  trig/1 -> trig_delay/1(d)
  trig_delay/1(q) -> ss/3(trig)

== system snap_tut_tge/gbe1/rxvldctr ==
  out_reg : Inport
  assert_reg : xbsIndex_r4/Assert  assert_type=on  type_source=Explicitly  gui_display_data_type=Fixed-point  arith_type=Unsigned  n_bits=32  bin_pt=0  preci_type=Single  exp_width=8  frac_width=24  assert_rate=off  rate_source=Explicitly  period=1  output_port=on  block_type=assert
  cast_gw : xbsIndex_r4/Convert  gui_display_data_type=Fixed-point  arith_type=Unsigned  n_bits=32  bin_pt=0  float_type=Single  exp_bits=8  fraction_bits=24  quantization=Truncate  overflow=Wrap  en=off  latency=1  pipeline=off  dbl_ovrd=off  block_type=convert
  io_delay : xbsIndex_r4/Delay  rst=off  infoeditControl=Selection of Reset will increase slice count due to use of real FFs and instead of SRLs  en=off  latency=1  reg_retiming=on  dbl_ovrd=off  block_type=delay
  reint1 : xbsIndex_r4/Reinterpret  force_arith_type=on  arith_type=Unsigned  force_bin_pt=on  bin_pt=0  block_type=reinterpret
  sim_out : Terminator
  snap_tut_tge_gbe1_rxvldctr_user_data_in : xbsIndex_r4/Gateway Out  inherit_from_input=off  hdl_port=on  rows=1  columns=1  UseAsDAC=off  DACChannel='1'  interface=None  automatic_assignment=on  address_offset=hex2dec('00')  intf_name=''  intf_description=''  timing_constraint=None  locs_specified=off  LOCs={}  io_standard={}  block_type=gatewayout
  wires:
  io_delay/1 -> cast_gw/1
  cast_gw/1 -> snap_tut_tge_gbe1_rxvldctr_user_data_in/1
  snap_tut_tge_gbe1_rxvldctr_user_data_in/1 -> sim_out/1
  out_reg/1 -> assert_reg/1
  assert_reg/1 -> reint1/1
  reint1/1 -> io_delay/1

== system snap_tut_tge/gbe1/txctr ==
  out_reg : Inport
  assert_reg : xbsIndex_r4/Assert  assert_type=on  type_source=Explicitly  gui_display_data_type=Fixed-point  arith_type=Unsigned  n_bits=32  bin_pt=0  preci_type=Single  exp_width=8  frac_width=24  assert_rate=off  rate_source=Explicitly  period=1  output_port=on  block_type=assert
  cast_gw : xbsIndex_r4/Convert  gui_display_data_type=Fixed-point  arith_type=Unsigned  n_bits=32  bin_pt=0  float_type=Single  exp_bits=8  fraction_bits=24  quantization=Truncate  overflow=Wrap  en=off  latency=1  pipeline=off  dbl_ovrd=off  block_type=convert
  io_delay : xbsIndex_r4/Delay  rst=off  infoeditControl=Selection of Reset will increase slice count due to use of real FFs and instead of SRLs  en=off  latency=1  reg_retiming=on  dbl_ovrd=off  block_type=delay
  reint1 : xbsIndex_r4/Reinterpret  force_arith_type=on  arith_type=Unsigned  force_bin_pt=on  bin_pt=0  block_type=reinterpret
  sim_out : Terminator
  snap_tut_tge_gbe1_txctr_user_data_in : xbsIndex_r4/Gateway Out  inherit_from_input=off  hdl_port=on  rows=1  columns=1  UseAsDAC=off  DACChannel='1'  interface=None  automatic_assignment=on  address_offset=hex2dec('00')  intf_name=''  intf_description=''  timing_constraint=None  locs_specified=off  LOCs={}  io_standard={}  block_type=gatewayout
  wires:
  io_delay/1 -> cast_gw/1
  cast_gw/1 -> snap_tut_tge_gbe1_txctr_user_data_in/1
  snap_tut_tge_gbe1_txctr_user_data_in/1 -> sim_out/1
  out_reg/1 -> assert_reg/1
  assert_reg/1 -> reint1/1
  reint1/1 -> io_delay/1
